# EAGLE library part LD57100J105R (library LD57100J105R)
Linear Voltage Regulator IC Positive Fixed 1 Output 1A 6-FlipChip (0.78x1.18) Source: Datasheet
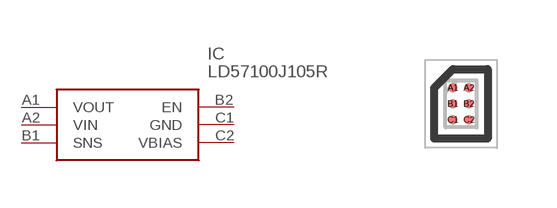
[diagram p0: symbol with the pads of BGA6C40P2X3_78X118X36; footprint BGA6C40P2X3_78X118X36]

Designator prefix IC

## LD57100J105R (Description: Linear Voltage Regulator IC Positive Fixed 1 Output 1A 6-FlipChip (0.78x1.18); Height: 0.361mm; Manufacturer_Name: STMicroelectronics; Manufacturer_Part_Number: LD57100J105R; Mouser_Part_Number: 511-LD57100J105R; Mouser_Price-Stock: https://www.mouser.co.uk/ProductDetail/STMicroelectronics/LD57100J105R?qs=TiOZkKH1s2SYSWW8899gzw%3D%3D)  [BGA6C40P2X3_78X118X36]
A1  VOUT
A2  VIN
B1  SNS
B2  EN
C1  GND
C2  VBIAS

## Footprint BGA6C40P2X3_78X118X36 (pad centres in mm)
Flip Chip6 (0.8x1.2 mm) package mechanical data
smd 0.234 x 0.234: A1 -0.2,0.4; A2 0.2,0.4; B1 -0.2,0; B2 0.2,0; C1 -0.2,-0.4; C2 0.2,-0.4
